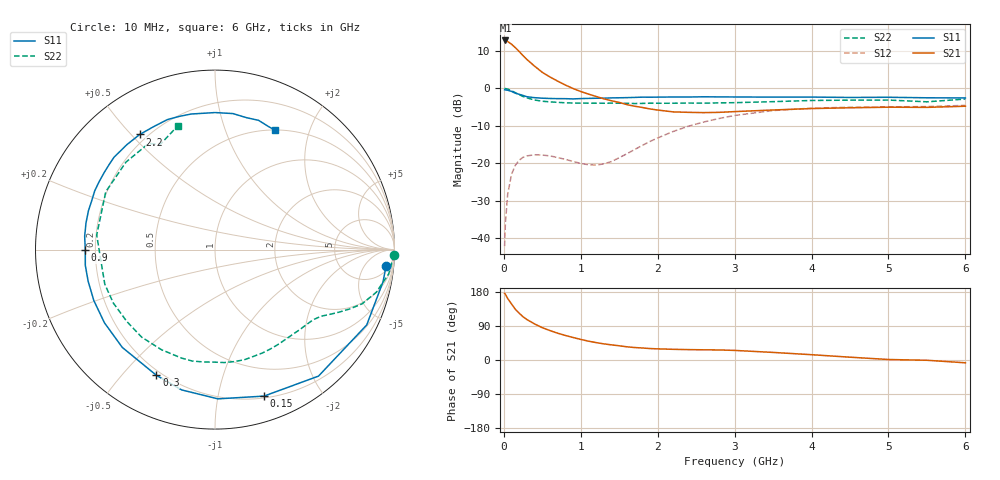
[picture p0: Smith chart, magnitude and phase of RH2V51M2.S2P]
! SIEMENS Small Signal Semiconductors
! BFR106
! Si NPN RF Bipolar Junction Transistor in SOT23
! VCE = 2.5 V  IC = 1.2 mA
! Common Emitter S-Parameters:  August  1996
# GHz  S  MA  R  50
!  f  S11  S21  S12  S22
! GHz  MAG  ANG  MAG  ANG  MAG  ANG  MAG  ANG
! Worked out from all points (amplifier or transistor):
!   36 points, 10 MHz to 6 GHz, reference 50 ohm
!   highest |S21| = 12.8 dB at 20 MHz (marker M1)
!   |S21| within 3 dB of that: start of sweep to 201.6 MHz
!   unconditionally stable (mu >= 1): 840.2 MHz to end of sweep
!   at 250 MHz: K = 0.27, MSG = 13.6 dB, |S12| = -18.4 dB
!   at 1.4 GHz: K = 1.42, MAG = 4.3 dB, |S12| = -19.5 dB
!   at 6 GHz: K = 1.02, MAG = -1.0 dB, |S12| = -4.6 dB
!   S11 on the Smith chart (normalised r, x): 10 MHz: 8, -17; 150 MHz: 0.22, -1.37; 300 MHz: 0.18, -0.62; 900 MHz: 0.16, -0.00; 2.2 GHz: 0.17, +0.53; 6 GHz: 0.50, +1.51
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0.01  0.9576 -5.5  4.358 175.8  0.0078 88.0  0.9989 -1.7
0.02  0.9533 -10.8  4.361 173.3  0.0157 84.7  0.9914 -3.3
0.05  0.9438 -26.4  4.221 162.4  0.0386 75.1  0.977 -8.0
0.1  0.9107 -50.7  3.888 147.8  0.0711 62.4  0.9295 -14.8
0.15  0.8607 -71.5  3.489 133.7  0.0942 50.6  0.8738 -20.2
0.2  0.8317 -88.9  3.1 123.5  0.1098 42.6  0.823 -23.6
0.25  0.8035 -103.4  2.731 114.0  0.1201 35.6  0.778 -26.5
0.3  0.7727 -115.0  2.428 106.8  0.1253 30.7  0.7463 -28.6
0.4  0.7508 -133.5  1.977 95.1  0.1297 23.3  0.6986 -32.1
0.5  0.7387 -146.5  1.636 85.3  0.1285 18.8  0.673 -35.4
0.7  0.7284 -166.0  1.248 70.7  0.1191 15.3  0.65 -43.1
0.9  0.7226 -179.7  0.995 59.4  0.1057 18.8  0.6364 -51.3
1.1  0.7339 168.3  0.838 49.7  0.0954 29.5  0.6339 -60.6
1.3  0.739 158.3  0.725 42.6  0.098 45.5  0.6325 -70.2
1.6  0.7517 145.4  0.606 34.8  0.1339 64.0  0.6315 -85.3
2.2  0.7664 123.2  0.485 28.2  0.2651 66.0  0.6325 -118.1
2.8  0.7684 105.0  0.478 26.5  0.3963 52.4  0.6399 -152.2
3.5  0.7635 90.0  0.514 20.0  0.505 34.6  0.664 173.0
4.5  0.7557 76.6  0.55 7.4  0.5595 13.4  0.6955 135.5
5  0.7601 71.4  0.56 1.3  0.5662 5.6  0.6974 122.0
5.5  0.7478 66.6  0.557 -0.7  0.5708 2.0  0.661 117.4
6  0.7445 63.2  0.577 -7.4  0.5922 -5.5  0.7194 106.8
